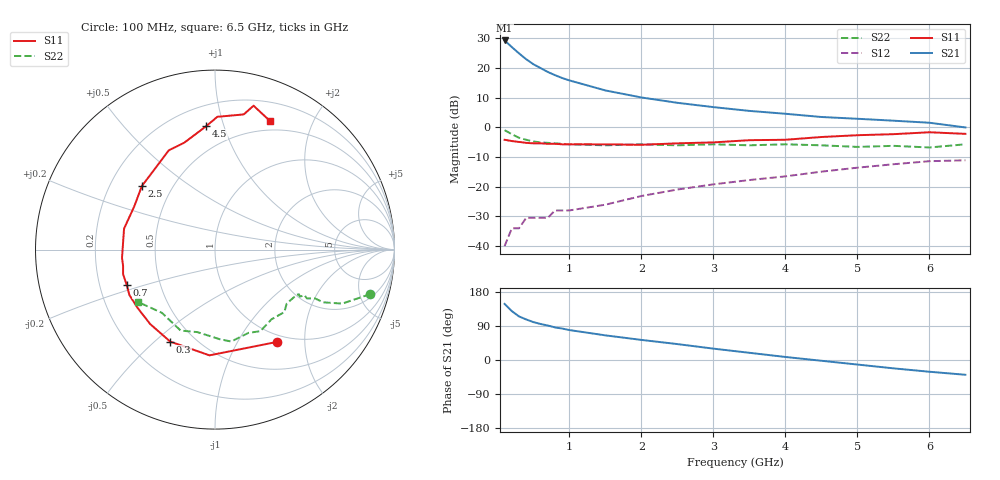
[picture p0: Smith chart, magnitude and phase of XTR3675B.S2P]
! HXTR-3675 Common Emitter
! Vce=15V  Ic=18mA
# ghz s ma r 50
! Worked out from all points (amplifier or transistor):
!   21 points, 100 MHz to 6.5 GHz, reference 50 ohm
!   highest |S21| = 29.3 dB at 100 MHz (marker M1)
!   |S21| within 3 dB of that: start of sweep to 236.5 MHz
!   unconditionally stable (mu >= 1): 1.146 GHz to 2.458 GHz
!   at 400 MHz: K = 0.46, MSG = 26.7 dB, |S12| = -30.5 dB
!   at 1.5 GHz: K = 1.15, MAG = 16.9 dB, |S12| = -26.0 dB
!   at 6.5 GHz: K = 0.50, MSG = 5.5 dB, |S12| = -11.1 dB
!   S11 on the Smith chart (normalised r, x): 100 MHz: 0.89, -1.49; 300 MHz: 0.37, -0.56; 700 MHz: 0.32, -0.18; 2.5 GHz: 0.34, +0.34; 4.5 GHz: 0.33, +0.88; 6.5 GHz: 0.39, +1.44
0.1  0.62 -56.0  29.2 148.0  0.01 69.0  0.9 -16.0
0.2  0.59 -93.0  22.6 129.0  0.02 66.0  0.77 -23.0
0.3  0.57 -116.0  17.7 115.0  0.02 50.0  0.67 -26.0
0.4  0.55 -131.0  14.1 107.0  0.03 55.0  0.62 -26.0
0.5  0.54 -143.0  11.6 100.0  0.03 47.0  0.58 -28.0
0.6  0.54 -152.0  10 95.0  0.03 48.0  0.56 -27.0
0.7  0.53 -158.0  8.6 91.0  0.03 51.0  0.55 -28.0
0.8  0.53 -165.0  7.6 86.0  0.04 52.0  0.54 -29.0
0.9  0.52 -170.0  6.8 83.0  0.04 57.0  0.53 -28.0
1  0.52 -175.0  6.2 79.0  0.04 57.0  0.52 -29.0
1.5  0.52 167.0  4.2 65.0  0.05 59.0  0.5 -37.0
2  0.51 152.0  3.2 53.0  0.07 63.0  0.52 -42.0
2.5  0.54 139.0  2.6 42.0  0.09 64.0  0.5 -51.0
3  0.56 127.0  2.2 30.0  0.11 62.0  0.52 -61.0
3.5  0.61 115.0  1.9 19.0  0.13 59.0  0.5 -68.0
4  0.62 106.0  1.7 8.0  0.15 55.0  0.52 -80.0
4.5  0.69 94.0  1.5 -2.0  0.18 51.0  0.5 -87.0
5  0.74 89.0  1.4 -12.0  0.21 45.0  0.47 -102.0
5.5  0.77 78.0  1.3 -22.0  0.24 38.0  0.49 -113.0
6  0.83 75.0  1.2 -31.0  0.27 34.0  0.46 -130.0
6.5  0.78 67.0  1 -39.0  0.28 28.0  0.52 -146.0
